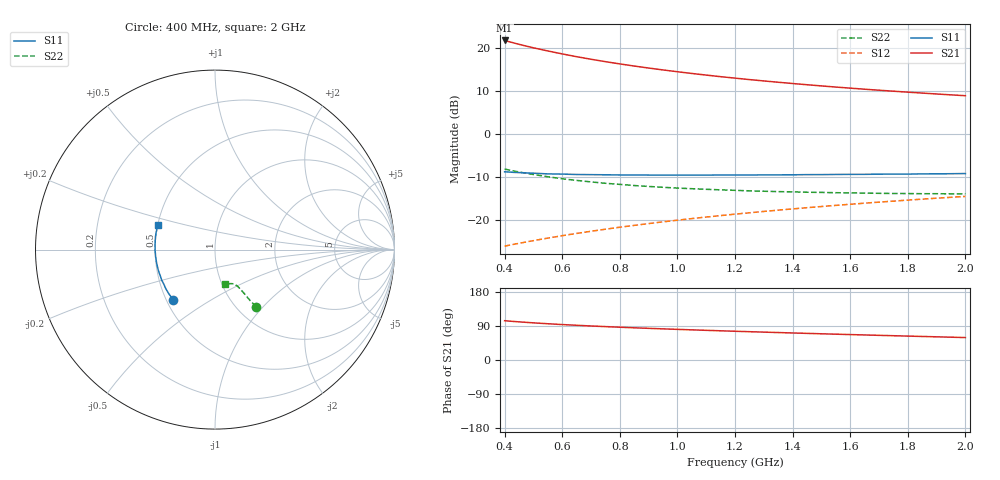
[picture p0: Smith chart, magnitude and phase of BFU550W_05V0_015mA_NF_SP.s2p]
! Filename:  P:\Prog\Test\Noise\ATS_data\Testdata_Net\06 Compressed Noise after Statistics\BFU550W_APM2013_11_D05_05p0V_015mA_NF_CM01_D.sf
! Date/Time: Tue 26/Mar/2013 16:25:24
! BFU550W_APM2013_11_D05_05p0V_1to35mA_NF_CM01_Bias7_R.sf
! Noise Parameter Data File
! BFU550W_APM2013_11_D05_05p0V_1to35mA_NF_CM01
! Date/time: Mon Mar 25 13:26:50 2013
! VAR V_out= 5.001000
! VAR I_out= 15.000000
! VAR V_in= 0.825200
! VAR I_in= 0.156650
! Device data file deembeded for feedlines and parallel
! Original file: \06 Compressed Noise after Statistics\BFU550W_APM2013_11_D05_05p0V_015mA_NF_CM01_R.sf
! Feed-files: PR019V01_070313_Feed1.s2p, PR019V01_070313_Feed2.s2p
! Parallel-file: PR019V01_070313_Par.s2p
# MHz S MA R 50
!  Freq-MHz  S11-mag  S11-arg  S21-mag  S21-arg  S12-mag  S12-arg  S22-mag  S22-arg
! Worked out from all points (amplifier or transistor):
!   37 points, 400 MHz to 2 GHz, reference 50 ohm
!   highest |S21| = 21.9 dB at 400 MHz (marker M1)
!   |S21| within 3 dB of that: start of sweep to 589.9 MHz
!   unconditionally stable (mu >= 1): 1.206 GHz to end of sweep
!   at 500 MHz: K = 0.84, MSG = 22.5 dB, |S12| = -24.8 dB
!   at 1.1 GHz: K = 0.99, MSG = 16.6 dB, |S12| = -19.3 dB
!   at 2 GHz: K = 1.01, MAG = 11.1 dB, |S12| = -14.5 dB
!   lowest NFmin = 0.81 dB at 400 MHz
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400  0.3644 -129.6  12.39 103.7  0.04939 62.5  0.3916 -54.1
420  0.3608 -132.2  11.87 102.4  0.05099 62.7  0.3795 -54.5
440  0.3578 -134.7  11.4 101.2  0.05257 63.0  0.3678 -54.8
460  0.3552 -136.9  10.96 100.1  0.05412 63.3  0.3573 -55.1
500  0.3504 -141.3  10.17 98.0  0.0573 63.8  0.3384 -55.5
550  0.3441 -145.9  9.345 95.7  0.06134 64.4  0.3187 -55.9
600  0.3422 -150.1  8.628 93.5  0.06542 64.9  0.3018 -56.2
650  0.3385 -153.8  8.011 91.6  0.06953 65.4  0.2889 -56.5
700  0.3372 -157.2  7.477 89.8  0.07371 65.8  0.2773 -56.9
750  0.336 -160.2  7.01 88.1  0.07788 66.2  0.2674 -57.1
800  0.3343 -163.3  6.598 86.5  0.0821 66.5  0.2596 -57.6
850  0.3341 -166.0  6.232 85.0  0.08631 66.7  0.2517 -57.7
950  0.3327 -170.6  5.611 82.2  0.09493 67.1  0.2401 -58.5
1050  0.3329 -174.8  5.106 79.5  0.1036 67.3  0.2312 -59.4
1150  0.3341 -178.9  4.685 77.1  0.1123 67.3  0.2241 -60.4
1200  0.3337 179.4  4.504 75.9  0.1167 67.2  0.2213 -61.1
1250  0.3339 177.6  4.331 74.7  0.121 67.2  0.2183 -61.5
1350  0.3353 174.5  4.032 72.4  0.13 67.0  0.2137 -62.8
1500  0.3375 169.9  3.654 69.2  0.1433 66.5  0.2092 -65.1
1650  0.34 165.7  3.345 66.1  0.1566 65.9  0.2054 -67.4
1750  0.342 163.3  3.171 64.1  0.1656 65.4  0.2031 -69.2
2000  0.3473 157.1  2.808 59.2  0.188 64.0  0.2009 -74.2
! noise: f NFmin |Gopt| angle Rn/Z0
400  0.8133  0.2158  -178.1  0.0698
460  0.8486  0.2197  -178.1  0.0662
600  0.8688  0.211  -170.3  0.0718
800  0.8906  0.2516  -172.5  0.0642
1000  0.9224  0.255  -168.8  0.0659
1200  0.9602  0.2768  -168.9  0.0638
1400  0.9992  0.29  -163.1  0.0669
1600  1.011  0.3068  -162.6  0.0665
1800  1.052  0.3273  -156.3  0.0679
2000  1.075  0.338  -154  0.0738
